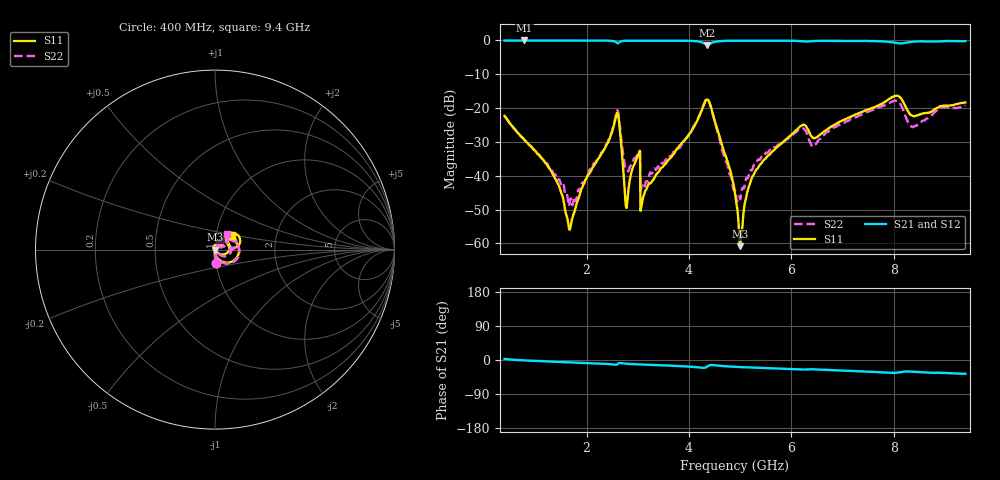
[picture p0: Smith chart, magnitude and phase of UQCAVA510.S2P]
!  Part Number  UQCAVA510	Mounting Orientation: Horizontal
!  Description: RF capacitors
!  Application: Coupling, Bypass, Tuning, DC Block
!  Filters, Matching
# GHZ S DB R 50
! Freq  |S11|  S11 Ph  |S21|  S21 Ph  |S12|  S12 Ph  |S22|  S22 Ph
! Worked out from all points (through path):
!   801 points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, 400 MHz to 9.4 GHz, reference 50 ohm
!   highest |S21| = -0.02 dB at 783 MHz (marker M1); lowest = -1.3 dB at 4.36 GHz (marker M2)
!   group delay of S21, straight-line fit = 11.3 ps
!   lowest |S11| = -60.8 dB at 5.001 GHz (marker M3), VSWR 1.00, Z = 50.1 - j0.0222 ohm
!   |S11| at or under -10 dB: start of sweep to end of sweep
!   |S22| runs from -48.9 to -17.2 dB; largest |S21 - S12| = 0.0028
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0.4  -22.29 -86.7  -0.04 2.9  -0.03 2.9  -22.33 -86.7
0.783  -29.30 -91.3  -0.02 -1.0  -0.01 -1.0  -29.32 -89.6
1.368  -40.25 -103.6  -0.03 -4.5  -0.02 -4.5  -39.57 -76.7
1.66  -55.80 -131.0  -0.04 -6.0  -0.02 -6.0  -48.93 -30.8
1.908  -43.74 106.2  -0.04 -7.2  -0.03 -7.2  -42.19 36.7
2.594  -21.49 26.5  -0.73 -11.8  -0.72 -11.9  -20.81 13.1
2.639  -24.56 -26.2  -0.57 -8.0  -0.56 -8.0  -23.41 -34.3
2.785  -49.48 38.3  -0.11 -9.9  -0.10 -9.9  -37.96 -4.7
2.999  -34.29 94.6  -0.07 -11.4  -0.06 -11.5  -33.39 51.5
3.1  -46.72 93.0  -0.06 -12.0  -0.05 -12.0  -42.93 12.8
3.404  -38.97 85.6  -0.07 -13.6  -0.06 -13.6  -37.29 42.9
4.36  -17.45 -6.7  -1.34 -17.3  -1.33 -17.3  -17.25 -12.9
4.9  -45.20 -87.8  -0.10 -17.9  -0.10 -18.0  -44.37 -39.2
5.001  -60.82 -14.1  -0.09 -18.6  -0.09 -18.6  -46.99 17.4
5.17  -43.21 73.1  -0.09 -19.6  -0.09 -19.6  -39.74 57.5
5.361  -37.41 73.6  -0.09 -20.6  -0.09 -20.6  -35.21 57.3
6.183  -25.32 55.4  -0.22 -25.1  -0.22 -25.2  -26.14 42.4
6.408  -28.60 38.3  -0.23 -24.5  -0.23 -24.5  -31.33 33.7
7.904  -17.38 43.9  -0.42 -33.5  -0.43 -33.6  -18.67 37.3
8.095  -16.49 20.6  -0.87 -32.9  -0.87 -33.0  -18.11 12.9
8.376  -22.37 20.3  -0.37 -31.1  -0.38 -31.2  -25.64 26.6
9.4  -18.34 38.4  -0.22 -36.3  -0.23 -36.4  -19.10 52.0
